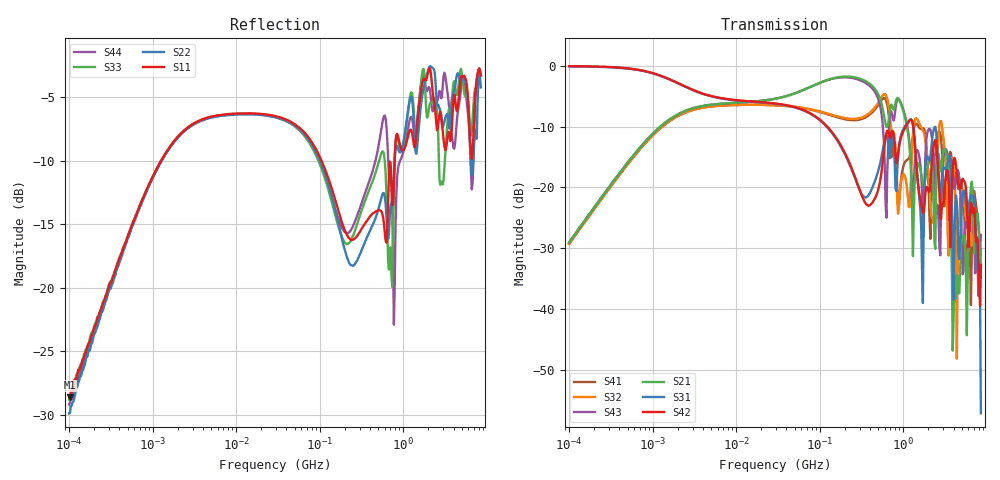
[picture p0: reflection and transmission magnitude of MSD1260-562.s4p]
# MHz S MA R 50
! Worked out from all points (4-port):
!   498 points, 100 kHz to 8.5 GHz, reference 50 ohm
!   strongest paths, dB at 100 kHz, 1.698 MHz, 29.49 MHz, 500.7 MHz, 8.5 GHz:
!     S42: -0.1, -2.4, -6.2, -20.4, -32.7
!     S31: -0.1, -2.4, -6.3, -17.3, -57.2
!     S21: -29.1, -8.6, -5.4, -4.7, -30.4
!     S43: -29.2, -8.6, -5.4, -5.4, -27.8
!     S32: -29.3, -8.8, -6.5, -6.1, -34.8
!     S41: -29.3, -8.8, -6.5, -6.5, -31.1
!   lowest |S11| = -28.6 dB at 102.3 kHz (marker M1), VSWR 1.08, Z = 50.2 + j3.71 ohm
!   |S11| at or under -10 dB: start of sweep to 1.264 MHz; 105 MHz to 789.1 MHz (684.1 MHz wide, 153 % of centre)
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0.1  0.03702 85.5  0.03525 84.3  0.9907 -2.1  0.03431 -96.4
     0.03525 84.3  0.03205 87.9  0.03411 -95.4  0.9932 -2.0
     0.9907 -2.1  0.03411 -95.4  0.03629 86.0  0.03484 84.3
     0.03431 -96.4  0.9932 -2.0  0.03484 84.3  0.0347 86.8
0.1023101  0.037 85.5  0.03598 84.1  0.9908 -2.2  0.0348 -96.0
           0.03598 84.1  0.03215 87.1  0.03508 -95.8  0.9928 -2.1
           0.9908 -2.2  0.03508 -95.8  0.03754 86.9  0.03598 83.6
           0.0348 -96.0  0.9928 -2.1  0.03598 83.6  0.03542 86.9
187.5231  0.1778 -46.0  0.8134 -25.9  0.2042 -117.2  0.367 63.1
          0.8134 -25.9  0.1523 -51.1  0.3746 59.4  0.209 -114.8
          0.2042 -117.2  0.3746 59.4  0.1564 -36.4  0.8027 -28.0
          0.367 63.1  0.209 -114.8  0.8027 -28.0  0.1702 -32.6
2365.873  0.525 155.2  0.03498 12.6  0.3125 121.5  0.1633 157.5
          0.03498 12.6  0.7098 157.5  0.06055 175.7  0.2352 118.0
          0.3125 121.5  0.06055 175.7  0.5583 167.1  0.1332 57.3
          0.1633 157.5  0.2352 118.0  0.1332 57.3  0.5317 173.0
4913.36  0.6723 -86.5  0.03297 -156.0  0.04572 -78.6  0.1149 -135.0
         0.03297 -156.0  0.6423 -95.2  0.08845 -88.5  0.1021 -119.5
         0.04572 -78.6  0.08845 -88.5  0.7257 -87.8  0.06167 82.7
         0.1149 -135.0  0.1021 -119.5  0.06167 82.7  0.6009 -81.2
6764.496  0.3402 66.6  0.09664 -2.6  0.085 21.0  0.06861 138.6
          0.09664 -2.6  0.2874 54.5  0.04013 -179.6  0.06169 32.3
          0.085 21.0  0.04013 -179.6  0.4667 60.8  0.07966 -32.7
          0.06861 138.6  0.06169 32.3  0.07966 -32.7  0.2582 100.4
8500  0.6841 -55.6  0.0303 -80.7  0.00138 -139.9  0.02797 -136.4
      0.0303 -80.7  0.6134 -45.3  0.0181 175.6  0.02305 -141.9
      0.00138 -139.9  0.0181 175.6  0.6804 -49.8  0.04055 -15.9
      0.02797 -136.4  0.02305 -141.9  0.04055 -15.9  0.6818 -51.9
